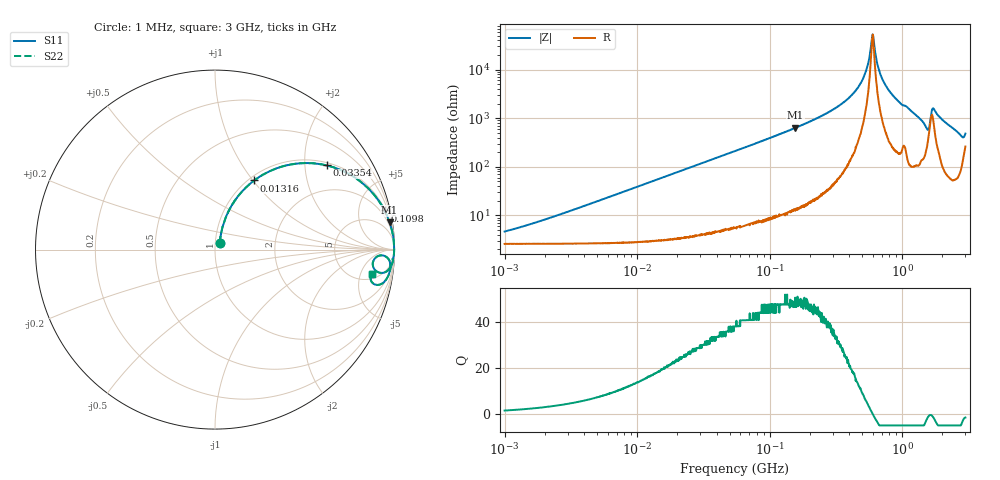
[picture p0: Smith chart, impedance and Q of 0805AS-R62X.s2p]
!s-Parameter Generated by FASTRON Sdn. Bhd.
!FASTRON P/N : 0805AS-R62X
!Keysight Technologies: E4991B_MY54100416_A.01.15
!Date: Mon Jun 15 12:55:35 2026
!Version  :Rev01  Mon Jun 15 12:55:35 2026
!Data & Calibration Information:
!Freq  S11  S21  S12  S22
!PortZ  Port1:50+j0  Port2:50+j0
!When reading reference impedance value at option line is always used.
! Remarks : This data is being provided solely for informational purposes.
# Hz S dB R 50
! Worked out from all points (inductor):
!   1601 points, 1 MHz to 3 GHz, reference 50 ohm
!   read as one part in series: L = 615 nH near 2.025 MHz
!   highest Q = 49 at 156.7 MHz (marker M1), where L = 646 nH
!   self-resonance near 598.9 MHz
!   S11 on the Smith chart (normalised r, x): 1 MHz: 1.05, +0.08; 13.16 MHz: 1.06, +1.02; 33.54 MHz: 1.08, +2.58; 109.8 MHz: 1.19, +8.62; 3 GHz: 6, -8
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1000000  -26.90 54.1  -0.23 -2.2  -0.23 -2.2  -26.90 54.1
3804036  -16.80 71.7  -0.31 -8.2  -0.31 -8.2  -16.80 71.7
1.315826e7  -7.07 60.4  -1.20 -26.2  -1.20 -26.2  -7.07 60.4
1.447069e7  -6.43 58.5  -1.38 -28.4  -1.38 -28.4  -6.43 58.5
3.354185e7  -2.17 37.1  -4.39 -51.1  -4.39 -51.1  -2.17 37.1
5.504702e7  -0.96 25.0  -7.48 -63.5  -7.48 -63.5  -0.96 25.0
1.098084e8  -0.27 13.0  -12.90 -75.8  -12.90 -75.8  -0.27 13.0
1.566509e8  -0.13 8.9  -16.20 -79.9  -16.20 -79.9  -0.13 8.9
2.083556e8  -0.07 6.4  -19.10 -82.4  -19.10 -82.4  -0.07 6.4
3.334925e8  -0.03 3.2  -25.20 -85.0  -25.20 -85.0  -0.03 3.2
4.480278e8  -0.02 1.5  -31.50 -84.7  -31.50 -84.7  -0.02 1.5
5.258324e8  -0.02 0.7  -38.50 -80.5  -38.50 -80.5  -0.02 0.7
5.840965e8  -0.02 0.1  -50.50 -50.2  -50.50 -50.2  -0.02 0.1
5.988949e8  -0.02 0.0  -54.50 -2.0  -54.50 -2.0  -0.02 0.0
6.140682e8  -0.02 -0.1  -50.50 49.1  -50.50 49.1  -0.02 -0.1
6.787043e8  -0.02 -0.7  -38.70 78.9  -38.70 78.9  -0.02 -0.7
7.925923e8  -0.02 -1.5  -31.50 83.4  -31.50 83.4  -0.02 -1.5
1.526649e9  -0.57 -8.0  -16.50 60.6  -16.50 60.6  -0.57 -8.0
1.581072e9  -1.05 -6.2  -16.30 38.8  -16.30 38.8  -1.05 -6.2
1.730092e9  -0.28 -3.1  -24.10 57.4  -24.10 57.4  -0.28 -3.1
2.75535e9  -0.53 -11.9  -13.60 67.8  -13.60 67.8  -0.53 -11.9
3e9  -1.03 -8.9  -14.70 48.3  -14.70 48.3  -1.03 -8.9
